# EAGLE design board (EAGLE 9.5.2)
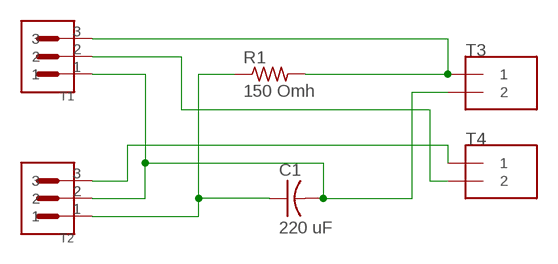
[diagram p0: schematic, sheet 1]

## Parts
C1  220 uF  CAP-US1206FAB  [C1206FAB]
R1  150 Omh  RES-US1206FAB  [R1206FAB]
T1  DG306-5.0-03P-12-00A(H)  [DEGSON_DG306-5.0-03P-12-00A(H)]
T2  DG306-5.0-03P-12-00A(H)  [DEGSON_DG306-5.0-03P-12-00A(H)]
T3  KF301-2P  [KF301-2P]
T4  KF301-2P  [KF301-2P]

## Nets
N$1: C1.1 R1.1 T2.1
N$2: R1.2 T1.3 T3.1
N$3: C1.2 T1.1 T2.2 T3.2
N$5: T2.3 T4.1
N$6: T1.2 T4.2

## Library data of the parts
C1 = fab:CAP-US
R1 = fab:RES-US: Resistor (US Symbol)
T1 T2 = DG306-5.0-03P-12-00A_H_:DG306-5.0-03P-12-00A(H): Terminal block; 5mm; angled 90°; 2.5mm2; ways: 3; tinned; 15A; blu; AVAILABILITY: Unavailable; DESCRIPTION: Terminal block; 5mm; angled 90°; 2.5mm2; ways: 3; tinned; 15A; blu; MF: Degson; MP: DG306-5.0-03P-12-00A(H); PACKAGE: None; PRICE: None
T3 T4 = KF301-2P:KF301-2P; AVAILABILITY: Unavailable; DESCRIPTION: 2 Pin Terminal Block 5mm Pitch; MF: Handson Technology; MP: KF301-2P; PACKAGE: Package Analog Devices; PRICE: None

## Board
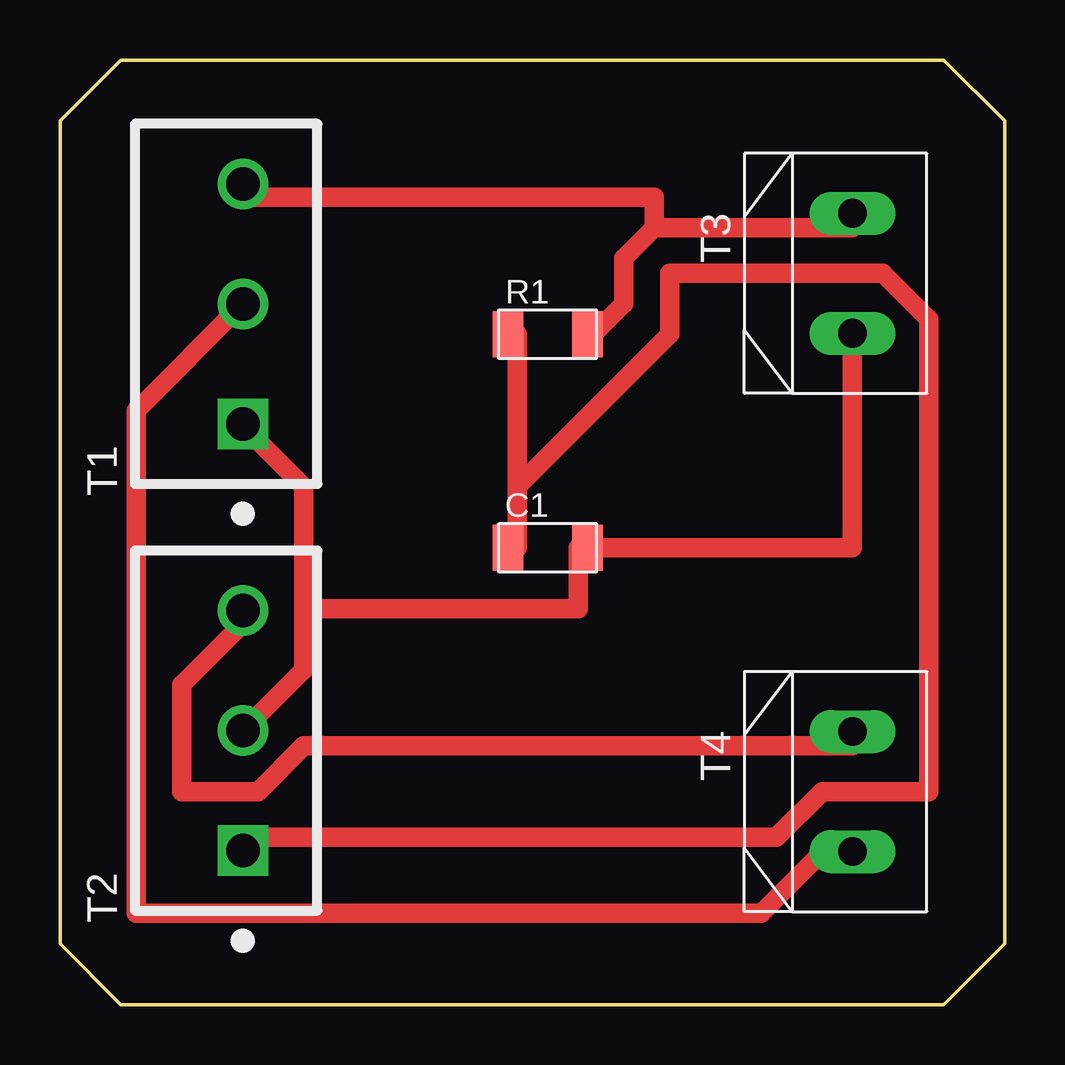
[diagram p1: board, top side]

Size 39.37 x 39.37 mm. Coordinates in mm from the lower left corner, seen from the top.
Outline: 0,2.54 0,36.83 2.54,39.37 36.83,39.37 39.37,36.83 39.37,2.54 36.83,0 2.54,0 0,2.54
Copper layers (1*16): Top 0.035mm / dielectric 1.5mm / Bottom 0.035mm
Design rules "default *": minimum track width 32mil, minimum drill 0.35mm, track to track 25mil, track to pad 25mil, pad to pad 6mil, via to via 6mil, smd to smd 6mil, copper to edge 40mil, drill to drill 6mil, minimum pad ring 10mil, minimum via ring 8mil, stop-mask expansion 4mil, vias tented up to drill 0mil, thermal gap 10mil

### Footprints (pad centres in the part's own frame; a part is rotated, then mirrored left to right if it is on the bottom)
C1206FAB = smd 1.27 x 1.905: 1 -1.651,0; 2 1.651,0
R1206FAB = smd 1.27 x 1.905: 1 -1.651,0; 2 1.651,0
DEGSON_DG306-5.0-03P-12-00A(H) = drill 1.4 square: 1 -5,0 | drill 1.4: 2 0,0; 3 5,0
KF301-2P = drill 1.2 pad 1.778 long: 1 -2.5,0; 2 2.5,0

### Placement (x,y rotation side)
C1  20.32,19.05 0 top
R1  20.32,27.94 0 top
T1  7.62,29.21 90 top
T2  7.62,11.43 90 top
T3  33.02,30.48 270 top
T4  33.02,8.89 270 top

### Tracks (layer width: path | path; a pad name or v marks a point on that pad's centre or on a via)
N$1
  Top 0.813: 19.05,21.59 19.05,27.94 R1.1 | 19.05,21.59 19.05,19.05 C1.1 | 19.05,21.59 25.4,27.94 25.4,30.48 34.29,30.48 36.2,28.57 36.2,8.89 31.75,8.89 29.84,6.99 7.62,6.99 T2.1
N$2
  Top 0.813: 24.77,32.38 23.5,31.11 23.5,29.21 22.23,27.94 R1.2 | 24.77,32.38 33.02,32.38 T3.1 | 24.77,32.38 24.77,33.65 7.62,33.65 T1.3
N$3
  Top 0.813: T2.2 10.16,13.97 10.16,16.51 | 10.16,16.51 10.16,21.59 7.62,24.13 T1.1 | T3.2 33.02,19.05 C1.2 21.59,19.05 21.59,16.51 10.16,16.51
N$5
  Top 0.813: T4.1 33.02,10.79 10.16,10.79 8.26,8.89 5.08,8.89 5.08,13.34 7.62,15.88 T2.3
N$6
  Top 0.813: T1.2 3.18,24.77 3.18,3.81 29.21,3.81 31.75,6.35 33.02,6.35 T4.2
